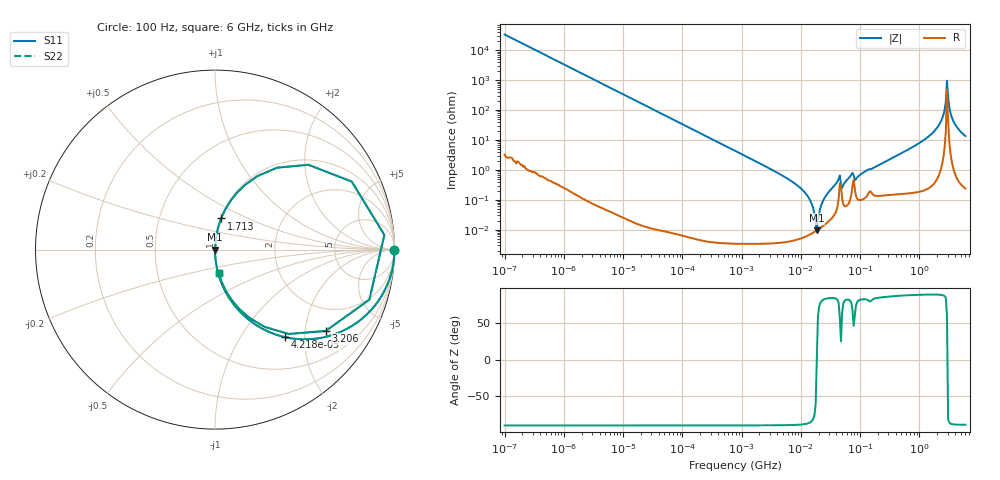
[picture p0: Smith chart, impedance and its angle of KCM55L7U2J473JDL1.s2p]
!Murata Part Number: KCM55L7U2J473JDL1
!These Parameters are Measured in Series Mode Connection
!Data Generated on Mar 13, 2026
!  o--ll--o
!Port1  Port2
!  o------o
!Operation Temp=25[degC], DC Bias Voltage=0[V]
!Freq. Start=100[Hz] Stop=6[GHz] 401[Steps]
# Hz S RI R 50
!Freq.(Hz) S11(Real) S11(Imag) S21(Real) S21(Imag) S12(Real) S12(Imag) S22(Real) S22(Imag)
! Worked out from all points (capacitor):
!   401 points, 100 Hz to 6 GHz, reference 50 ohm
!   read as one part in series: C = 47 nF near 109 Hz
!   lowest |Z| = 9.45 mohm at 18.61 MHz (marker M1)
!   series resonance near 18.6 MHz, so ESL is about 1.6 nH
!   S11 on the Smith chart (normalised r, x): 100 Hz: open; 42.18 kHz: 1.00, -1.61; 1.713 GHz: 1.01, +0.36; 3.206 GHz: 1.18, -2.57; 6 GHz: 1.00, -0.27
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100  1 -0.00295  9e-06 0.00295  9e-06 0.00295  1 -0.00295
2008  0.9965 -0.0591  0.00351 0.0591  0.00351 0.0591  0.9965 -0.0591
12041  0.8878 -0.3156  0.1122 0.3156  0.1122 0.3156  0.8878 -0.3156
40335  0.4136 -0.4924  0.5864 0.4924  0.5864 0.4924  0.4136 -0.4924
42182  0.3921 -0.4882  0.6079 0.4882  0.6079 0.4882  0.3921 -0.4882
123542  0.07 -0.255  0.93 0.255  0.93 0.255  0.07 -0.255
774597  0.00194 -0.0436  0.9981 0.0436  0.9981 0.0436  0.00194 -0.0436
7599586  5.71e-05 -0.00372  0.9999 0.00372  0.9999 0.00372  5.71e-05 -0.00372
1.555665e7  7.65e-05 -0.000659  0.9999 0.000659  0.9999 0.000659  7.65e-05 -0.000659
1.86079e7  9.45e-05 1.4e-06  0.9999 -1.4e-06  0.9999 -1.4e-06  9.45e-05 1.4e-06
2.434276e7  0.000139 0.00101  0.9999 -0.00101  0.9999 -0.00101  0.000139 0.00101
4.165952e7  0.000623 0.0041  0.9994 -0.0041  0.9994 -0.0041  0.000623 0.0041
5.211241e7  0.000721 0.00302  0.9993 -0.00302  0.9993 -0.00302  0.000721 0.00302
7.129496e7  0.00153 0.00669  0.9985 -0.00669  0.9985 -0.00669  0.00153 0.00669
8.918374e7  0.00113 0.00544  0.9989 -0.00544  0.9989 -0.00544  0.00113 0.00544
3.124326e8  0.00194 0.0221  0.9981 -0.0221  0.9981 -0.0221  0.00194 0.0221
1.712697e9  0.0344 0.1736  0.9656 -0.1736  0.9656 -0.1736  0.0344 0.1736
2.562649e9  0.3459 0.4564  0.6541 -0.4564  0.6541 -0.4564  0.3459 0.4564
2.931063e9  0.9436 0.0816  0.0564 -0.0816  0.0564 -0.0816  0.9436 0.0816
3.205649e9  0.6168 -0.4533  0.3832 0.4533  0.3832 0.4533  0.6168 -0.4533
3.8344e9  0.1413 -0.3364  0.8587 0.3364  0.8587 0.3364  0.1413 -0.3364
6e9  0.0203 -0.1324  0.9797 0.1324  0.9797 0.1324  0.0203 -0.1324
